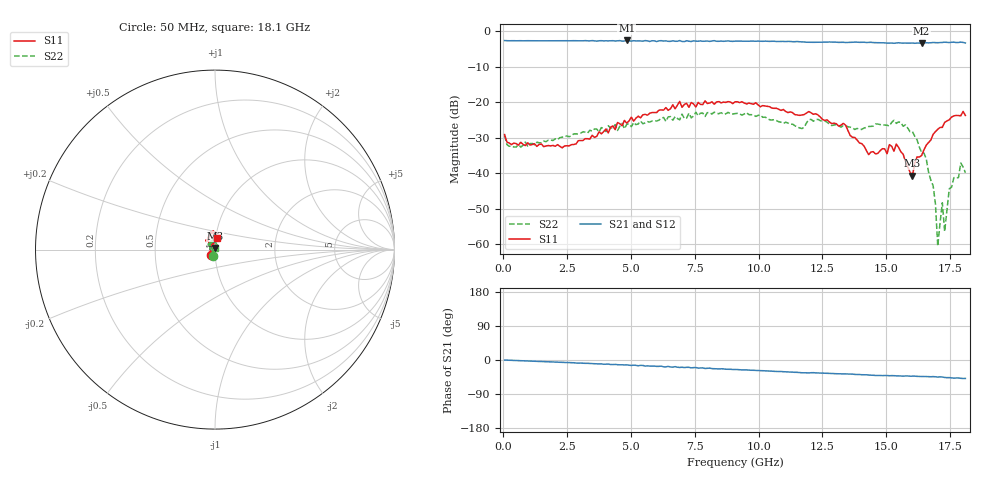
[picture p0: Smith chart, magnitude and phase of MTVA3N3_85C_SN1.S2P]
! Network Analyzer HP8720D.06.14 Serial No. US36140669
! 27 Jun 2005  08:49:56
! Frequency  S11  S21  S12  S22
# HZ  S  DB R 50
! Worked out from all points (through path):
!   201 points, 50 MHz to 18.1 GHz, reference 50 ohm
!   highest |S21| = -2.67 dB at 4.833 GHz (marker M1); lowest = -3.5 dB at 16.39 GHz (marker M2)
!   group delay of S21, straight-line fit = 7.5 ps
!   lowest |S11| = -40.7 dB at 16.02 GHz (marker M3), VSWR 1.02, Z = 50.1 + j0.919 ohm
!   |S11| at or under -10 dB: start of sweep to end of sweep
!   |S22| runs from -60.6 to -22.8 dB; largest |S21 - S12| = 0.02
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5e7  -29.17 -127.6  -2.70 -0.1  -2.73 0.2  -29.39 -104.3
6.8175e8  -31.32 174.9  -2.74 -1.8  -2.76 -1.7  -32.68 178.5
3.1185e9  -30.83 118.9  -2.77 -8.4  -2.78 -8.6  -28.36 142.1
4.83325e9  -25.93 101.0  -2.67 -12.8  -2.71 -13.5  -26.25 113.4
6.09675e9  -22.29 93.2  -2.77 -16.8  -2.73 -16.7  -25.10 96.5
9.075e9  -19.93 101.3  -2.86 -25.0  -2.84 -25.1  -23.25 65.8
1.21435e10  -23.45 131.1  -3.19 -33.4  -3.15 -33.6  -25.39 102.2
1.331675e10  -26.00 128.5  -3.19 -36.8  -3.21 -37.0  -26.64 116.1
1.43095e10  -34.80 134.1  -3.21 -39.6  -3.17 -39.8  -26.87 142.1
1.512175e10  -31.99 88.9  -3.41 -41.4  -3.35 -41.1  -26.75 138.2
1.53925e10  -31.84 61.7  -3.38 -41.9  -3.32 -41.4  -26.02 130.7
1.602425e10  -40.72 86.2  -3.39 -42.5  -3.47 -43.7  -28.31 84.1
1.638525e10  -35.02 101.0  -3.47 -43.3  -3.33 -43.3  -34.20 51.7
1.68365e10  -29.09 110.7  -3.26 -43.8  -3.20 -44.9  -43.56 -3.9
1.692675e10  -28.34 112.6  -3.29 -44.3  -3.22 -44.2  -48.66 -0.4
1.7017e10  -27.68 104.5  -3.30 -45.0  -3.38 -45.8  -60.56 115.3
1.71975e10  -27.12 101.0  -3.23 -44.9  -3.22 -44.0  -48.35 18.8
1.728775e10  -25.74 99.8  -3.16 -46.1  -3.10 -46.1  -56.44 179.9
1.746825e10  -25.00 91.5  -3.25 -46.4  -3.31 -46.3  -44.42 93.2
1.782925e10  -23.83 87.7  -3.24 -47.5  -3.23 -47.3  -41.25 93.5
1.79195e10  -23.86 86.2  -3.13 -48.4  -3.03 -47.7  -37.15 100.4
1.81e10  -23.78 82.4  -3.38 -48.6  -3.37 -49.5  -39.88 84.8
